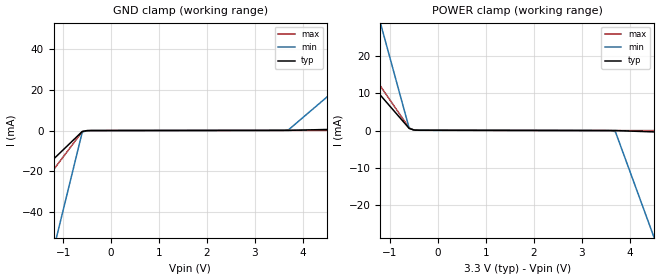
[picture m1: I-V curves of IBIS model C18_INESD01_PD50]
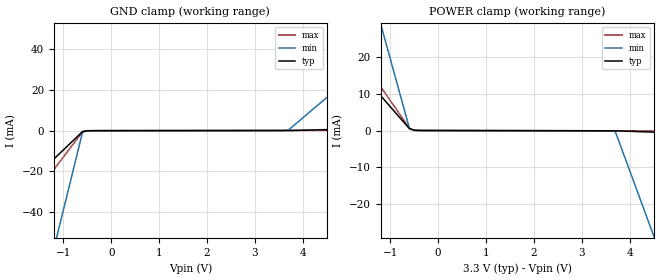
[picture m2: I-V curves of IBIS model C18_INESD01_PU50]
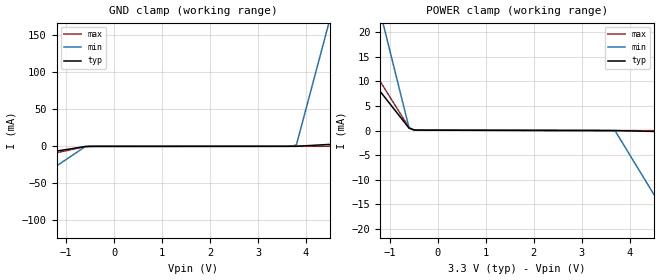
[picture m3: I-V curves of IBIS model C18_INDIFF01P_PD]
|   This file is an IBIS representation of the   |
|   Integrated Device Technology, Inc   |
|   ICS849N2505I   |
|   FEMTOCLOCK NG CLOCK SYNTHESIZER   |
[IBIS Ver]   4.1
[File name]   849n2505i_3v3.ibs
[File Rev]   1.0
[Date]   15 Sep 2009 | Last modified
[Source]   Originated at Integrated Device Technology, Inc.
[Disclaimer]
IDT hereby grants the user of this IBIS model a non-exclusive,
nontransferable license to use this IBIS model under the following terms.
Before using this IBIS model, the user should read this license.
If the user does not accept these terms,  the IBIS model should be
returned to IDT within 30 days.
   The user is granted this license only to use the IBIS model and
is not granted rights to sell, load, rent, lease or license the IBIS
model in whole or in part, or in modified form to anyone other than
user. User may modify the IBIS model to suit its specific
applications but rights to derivative works and such modifications
shall belong to IDT.
   This IBIS model is provided on an "AS IS" basis and IDT makes
absolutely no warranty with respect to the information contained
herein. IDT DISCLAIMS AND CUSTOMER WAIVES ALL WARRANTIES, EXPRESS
OR IMPLIED, INCLUDING WARRANTIES OF MERCHANTABILITY OR FITNESS FOR
A PARTICULAR PURPOSE. The entire risk as to quality and performance
is with the Customer. ACCORDINGLY, IN NO EVENT SHALL THE COMPANY BE
LIABLE FOR ANY DAMAGES, WHETHER IN CONTRACT OR TORT,INCLUDING ANY
LOST PROFITS OR OTHER INCIDENTAL, CONSEQUENTIAL, EXEMPLARY, OR
PUNITIVE DAMAGES ARISING OUT OF THE USE OR APPLICATION OF THE IBIS
model provided in this package. Further, IDT reserves the right to
make changes without notice to any product herein to improve
reliability, function, or design. IDT does not convey any license
under patent rights or any other intellectual property rights,
including those of third parties.
   IDT is not obligated to provide maintenance or support
for the licensed IBIS model.
[Copyright]   Copyright 2006 by Integrated Device Technology, Inc.
[Component]   ICS849N2505KI
[Manufacturer] Integrated Device Technology, Inc.
[Package]
|QFN 32LD
|lead + wire   typ   min   max
R_pkg   72.4655m   58.886m   86.045m
L_pkg   1.47175nH   1.11650nH   1.77850nH
C_pkg   0.07747pF   0.07444pF   0.08050pF
[Pin] signal_name   model_name   R_pin   L_pin   C_pin
1   PLL_BYPASS   C18_INESD01_PD50   86.045m   1.77850nH   0.08050pF
2   OE_REF   C18_INESD01_PD50   76.996m   1.55783nH   0.07848pF
3   OE1   C18_INESD01_PU50   67.941m   1.33717nH   0.07646pF
4   OE0   C18_INESD01_PU50   58.886m   1.11650nH   0.07444pF
5   LVDS_OUT   C18_INESD01_PD50   58.886m   1.11650nH   0.07444pF
6   VDDO_REF   POWER   67.941m   1.33717nH   0.07646pF
7   CLK   C18_INDIFF01P_PD   76.996m   1.55783nH   0.07848pF
8   nCLK   C18_INDIFF01N_PD   86.045m   1.77850nH   0.08050pF
9   REF_OUT   C18_OHSUNIV01_OE   86.045m   1.77850nH   0.08050pF
10  nREF_OUT   C18_OHSUNIV01_OE   76.996m   1.55783nH   0.07848pF
11  CLK_SEL   C18_INESD01_PU50   67.941m   1.33717nH   0.07646pF
12  XTAL_IN   NC   58.886m   1.11650nH   0.07444pF
13  XTAL_OUT   NC   58.886m   1.11650nH   0.07444pF
14  VDD   POWER   67.941m   1.33717nH   0.07646pF
15  FSEL0   C18_INESD01_PD50   76.996m   1.55783nH   0.07848pF
16  FSEL1   C18_INESD01_PD50   86.045m   1.77850nH   0.08050pF
17  nQ3   C18_OHSUNIV01_OE   86.045m   1.77850nH   0.08050pF
18  Q3   C18_OHSUNIV01_OE   76.996m   1.55783nH   0.07848pF
19  GND   GND   67.941m   1.33717nH   0.07646pF
20  nQ2   C18_OHSUNIV01_OE   58.886m   1.11650nH   0.07444pF
21  Q2   C18_OHSUNIV01_OE   58.886m   1.11650nH   0.07444pF
22  VDD   POWER   67.941m   1.33717nH   0.07646pF
23  nQ1   C18_OHSUNIV01_OE   76.996m   1.55783nH   0.07848pF
24  Q1   C18_OHSUNIV01_OE   86.045m   1.77850nH   0.08050pF
25  GND   GND   86.045m   1.77850nH   0.08050pF
26  nQ0   C18_OHSUNIV01_OE   76.996m   1.55783nH   0.07848pF
27  Q0   C18_OHSUNIV01_OE   67.941m   1.33717nH   0.07646pF
28  VDD   POWER   58.886m   1.11650nH   0.07444pF
29  OE3   C18_INESD01_PU50   58.886m   1.11650nH   0.07444pF
30  OE2   C18_INESD01_PU50   67.941m   1.33717nH   0.07646pF
31  VDD   POWER   76.996m   1.55783nH   0.07848pF
32  VDDA   POWER   86.045m   1.77850nH   0.08050pF
[Diff Pin]  inv_pin  vdiff tdelay_typ tdelay_min  tdelay_max
7   8   0.15   0   0   0
18   17   NA   0   0   0
21   20   NA   0   0   0
24   23   NA   0   0   0
27   26   NA   0   0   0
[Model Selector] C18_OHSUNIV01_OE
C18_LVDS_OHSUNIV   3.3V LVDS Driver
C18_LVPECL_OHSUN   3.3V LVPECL Driver
| Models and submodels in the file (6): C18_INESD01_PD50 (Input), C18_INESD01_PU50 (Input), C18_INDIFF01P_PD (Input), C18_INDIFF01N_PD (Input), C18_LVPECL_OHSUN (Output_ECL), C18_LVDS_OHSUNIV (Output)
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[Model]   C18_INESD01_PD50
Model_type   Input
Polarity   Non-Inverting
Vinl = 0.8V
Vinh = 2.2V
|   typ   min   max
C_comp   2pF   1.5pF   2.5pF
|   typ   min   max
[Voltage range]   3.3V   3.135V   3.465V
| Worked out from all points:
|   GND clamp passes 1 mA (typ) near -0.62 V on its own axis
|   POWER clamp passes 1 mA (typ) near -0.63 V on its own axis
[GND_clamp]
|Voltage   I (typ)   I (min)   I (max)
-3.3V     -61.32mA   -259.6mA   -84.4mA
-2.9V     -52.31mA   -221.3mA   -71.97mA
-2.8V     -50.05mA   -211.7mA   -68.87mA
-2.3V     -38.78mA   -163.7mA   -53.33mA
-2.2V     -36.52mA   -154.1mA   -50.23mA
-1.2V     -13.98mA   -58.24mA   -19.17mA
-1.1V     -11.73mA   -48.65mA   -16.06mA
-600mV    -453.3uA   -698.6uA   -527.7uA
-400mV    -11.1uA    -13uA      -9.761uA
3.7V      77.31uA    339.6uA    78.55uA
6.2V      1.427mA    50.43mA    134.4uA
6.6V      1.643mA    58.44mA    143.4uA
[Power_clamp]
|Voltage   I (typ)   I (min)   I (max)
-3.3V     40.74mA    127.9mA    51.33mA
-2.5V     28.83mA    90.18mA    36.32mA
-2.4V     27.35mA    85.47mA    34.44mA
-2.1V     22.88mA    71.33mA    28.82mA
-2V       21.4mA     66.62mA    26.94mA
-1.2V     9.494mA    28.91mA    11.94mA
-1.1V     8.006mA    24.2mA     10.06mA
-600mV    567.9uA    633.8uA    683uA
-500mV    131.3uA    131.4uA    134.2uA
3.7V      -11.1uA    -299.6uA   -4.991uA
4.5V      -367.9uA   -28.5mA    -22.78uA
6.6V      -1.304mA   -102.5mA   -69.48uA
[Model]   C18_INESD01_PU50
Model_type   Input
Polarity   Non-Inverting
Vinl = 0.8V
Vinh = 2.2V
|   typ   min   max
C_comp   2pF   1.5pF   2.5pF
|   typ   min   max
[Voltage range]   3.3V   3.135V   3.465V
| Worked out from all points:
|   GND clamp passes 1 mA (typ) near -0.62 V on its own axis
|   POWER clamp passes 1 mA (typ) near -0.63 V on its own axis
[GND_clamp]
|Voltage   I (typ)   I (min)   I (max)
-3.3V     -61.39mA   -259.7mA   -84.47mA
-2.9V     -52.37mA   -221.3mA   -72.05mA
-2.8V     -50.12mA   -211.7mA   -68.94mA
-2.3V     -38.84mA   -163.8mA   -53.41mA
-2.2V     -36.59mA   -154.2mA   -50.3mA
-1.2V     -14.05mA   -58.3mA    -19.24mA
-1.1V     -11.79mA   -48.71mA   -16.13mA
-600mV    -519.3uA   -757.2uA   -601.3uA
-400mV    -77.06uA   -71.62uA   -83.32uA
3.7V      11.34uA    280.9uA    4.99uA
6.2V      1.361mA    50.37mA    60.87uA
6.6V      1.577mA    58.38mA    69.81uA
[Power_clamp]
|Voltage   I (typ)   I (min)   I (max)
-3.3V     40.67mA    127.8mA    51.25mA
-2.5V     28.77mA    90.12mA    36.25mA
-2.4V     27.28mA    85.41mA    34.37mA
-2.1V     22.82mA    71.27mA    28.74mA
-2V       21.33mA    66.56mA    26.87mA
-1.2V     9.428mA    28.85mA    11.86mA
-1.1V     7.94mA     24.14mA    9.988mA
-600mV    501.9uA    575.2uA    609.4uA
-500mV    65.34uA    72.75uA    60.6uA
3.7V      -77.06uA   -358.2uA   -78.55uA
4.5V      -433.9uA   -28.56mA   -96.35uA
6.6V      -1.37mA    -102.6mA   -143uA
[Model]   C18_INDIFF01P_PD
Model_type   Input
Polarity   Non-Inverting
Vinl = 0.8V
Vinh = 2.2V
|   typ   min   max
C_comp   2pF   1.5pF   2.5pF
|   typ   min   max
[Voltage range]   3.3V   3.135V   3.465V
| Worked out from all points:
|   GND clamp passes 1 mA (typ) near -0.68 V on its own axis
|   POWER clamp passes 1 mA (typ) near -0.64 V on its own axis
[GND_clamp]
|Voltage   I (typ)   I (min)   I (max)
-3.3V     -27.91mA   -118mA     -38.4mA
-600mV    -212.6uA   -323.7uA   -246.8uA
3.6V      72.06uA    90.37uA    76.43uA
3.8V      122.1uA    1.964mA    80.77uA
4.4V      2.307mA    148.1mA    123uA
4.5V      2.671mA    172.4mA    130.1uA
6.6V      10.32mA    683.8mA    277.9uA
[Power_clamp]
|Voltage   I (typ)   I (min)   I (max)
-3.3V     33.97mA    106.6mA    42.8mA
-2.3V     21.57mA    67.31mA    27.16mA
-2.2V     20.33mA    63.39mA    25.6mA
-2V       17.85mA    55.53mA    22.47mA
-1.9V     16.61mA    51.6mA     20.91mA
-1.2V     7.927mA    24.11mA    9.964mA
-1.1V     6.687mA    20.18mA    8.4mA
-600mV    486.2uA    539.8uA    583.5uA
-500mV    122.1uA    120.8uA    125.8uA
3.7V      -9.408uA   -141.9uA   -4.99uA
5V        -287.1uA   -20.99mA   -33.19uA
6.6V      -628.9uA   -46.65mA   -67.89uA
